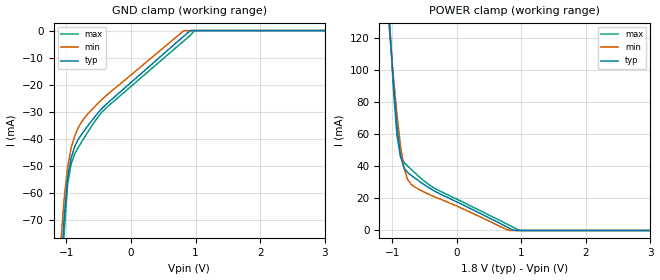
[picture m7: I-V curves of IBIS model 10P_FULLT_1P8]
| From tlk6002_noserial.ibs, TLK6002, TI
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[Model]   10P_FULLT_1P8
Model_type   Input
Polarity   Non-Inverting
Vinh =  1
Vinl =  0.8
C_comp   1.885425p   1.715283p   2.176444p
[Model Spec]
Vinh   1   0.91   1.09
Vinl   0.8   0.71   0.89
[Temperature Range]   25   125   -40
[Voltage Range]   1.8   1.62   1.98
[POWER_clamp]
-1.8V     664.6mA    540.3mA    800.7mA
-1.091V   158.9mA    148.6mA    170.4mA
-1.036V   124.2mA    121.5mA    127.4mA
-981.8mV  92.13mA    95.91mA    88.54mA
-927.3mV  64.9mA     72.58mA    59.15mA
-872.7mV  46.65mA    52.98mA    46.15mA
-818.2mV  39mA       39.16mA    42.51mA
-763.6mV  36.26mA    31.92mA    40.28mA
-654.5mV  32.86mA    27.2mA     36.13mA
763.6mV   2.439mA    687.8uA    4.272mA
981.8mV   0A         0A         0A
3.6V      0A         0A         0A
[GND_clamp]
-1.8V     -598.5mA   -433.2mA   -794.3mA
-1.091V   -93.44mA   -79.29mA   -108.8mA
-1.036V   -69.3mA    -62.34mA   -75.19mA
-981.8mV  -54.41mA   -50.46mA   -56.76mA
-927.3mV  -47.03mA   -43.33mA   -49.26mA
-872.7mV  -42.86mA   -38.98mA   -45.56mA
-818.2mV  -40.2mA    -35.92mA   -43.21mA
-709.1mV  -36.46mA   -31.91mA   -38.98mA
-381.8mV  -27.18mA   -23.96mA   -28.48mA
818.2mV   -2.072mA   0A         -3.831mA
981.8mV   0A         0A         0A
3.6V      0A         0A         0A
